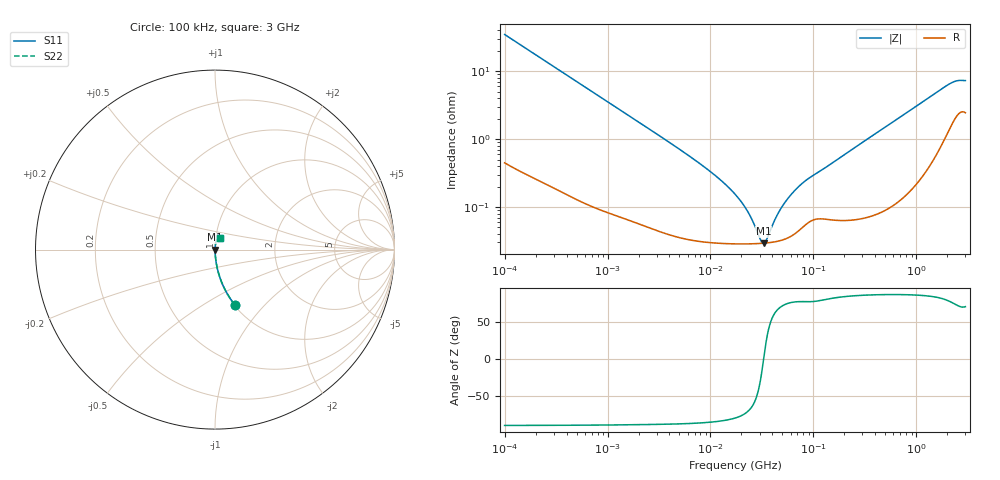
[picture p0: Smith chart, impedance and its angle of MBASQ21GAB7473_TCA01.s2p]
! MBASQ21GAB7473_TCA01  S-PARAMETER MODEL  ( Standard Model )
! Model Generated by TAIYO YUDEN Corporation (http://www.ty-top.com)
! Version 1.0
! TAIYO YUDEN Control No. 220601
! Copyright(c) 2022 TAIYO YUDEN CO.,LTD. All Rights Reserved.
! Product Description (link to TY-COMPAS)
! https://ds.yuden.co.jp/TYCOMPAS/or/detail?pn=MBASQ21GAB7473KTCA01&u=M
! Products Name : Multilayer Ceramic Capacitors
! Characteristics :
!  Capacitance : 0.047 [uF] , Rated Voltage : 250 [V] , TCC : X7R
!  Case Size : 2.0 x 1.25 / 0.079 x 0.049 [mm/inch] , Thickness : 1.25 / 0.049 [mm/inch]
!  (Conditions: Temperature = 25 [degC] , DC Bias Voltage = 0 [V])
! External Node Assignments :
!  1  o---| |---o  2
! GND o---------o GND
! Frequency Range : 100kHz  -  3GHz  [ 401 STEP ]
# MHZ S RI R 50
! Freq[MHz].  S11 Real  S11 Imag  S21 Real  S21 Imag  S12 Real  S12 Imag  S22 Real  S22 Imag
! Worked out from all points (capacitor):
!   401 points, 100 kHz to 3 GHz, reference 50 ohm
!   read as one part in series: C = 45.5 nF near 105.3 kHz
!   lowest |Z| = 29.3 mohm at 32.99 MHz (marker M1)
!   series resonance near 32.85 MHz, so ESL is about 520 pH
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0.1  0.1119 -0.3089  0.8881 0.3089  0.8881 0.3089  0.1119 -0.3089
0.147195  0.0563 -0.2238  0.9437 0.2238  0.9437 0.2238  0.0563 -0.2238
0.228123  0.0254 -0.1498  0.9746 0.1498  0.9746 0.1498  0.0254 -0.1498
0.562235  0.00512 -0.0626  0.9949 0.0626  0.9949 0.0626  0.00512 -0.0626
3.161081  0.000565 -0.0113  0.9994 0.0113  0.9994 0.0113  0.000565 -0.0113
9.574722  0.000312 -0.00348  0.9997 0.00348  0.9997 0.00348  0.000312 -0.00348
13.7349  0.000294 -0.00219  0.9997 0.00219  0.9997 0.00219  0.000294 -0.00219
17.7727  0.000288 -0.00145  0.9997 0.00145  0.9997 0.00145  0.000288 -0.00145
22.99754  0.000287 -0.000811  0.9997 0.000811  0.9997 0.000811  0.000287 -0.000811
25.49486  0.000287 -0.000571  0.9997 0.000571  0.9997 0.000571  0.000287 -0.000571
30.53531  0.00029 -0.000163  0.9997 0.000163  0.9997 0.000163  0.00029 -0.000163
32.15051  0.000292 -4.79e-05  0.9997 4.79e-05  0.9997 4.79e-05  0.000292 -4.79e-05
32.98988  0.000293 9.69e-06  0.9997 -9.69e-06  0.9997 -9.69e-06  0.000293 9.69e-06
34.73492  0.000295 0.000125  0.9997 -0.000125  0.9997 -0.000125  0.000295 0.000125
43.80277  0.00031 0.000656  0.9997 -0.000656  0.9997 -0.000656  0.00031 0.000656
53.83243  0.00034 0.00116  0.9997 -0.00116  0.9997 -0.00116  0.00034 0.00116
71.47675  0.000445 0.00193  0.9996 -0.00193  0.9996 -0.00193  0.000445 0.00193
97.38194  0.000642 0.00279  0.9994 -0.00279  0.9994 -0.00279  0.000642 0.00279
547.5153  0.00124 0.0165  0.9988 -0.0165  0.9988 -0.0165  0.00124 0.0165
2038.117  0.0163 0.0604  0.9837 -0.0604  0.9837 -0.0604  0.0163 0.0604
2441.062  0.0253 0.0657  0.9747 -0.0657  0.9747 -0.0657  0.0253 0.0657
3000  0.0283 0.0652  0.9717 -0.0652  0.9717 -0.0652  0.0283 0.0652
